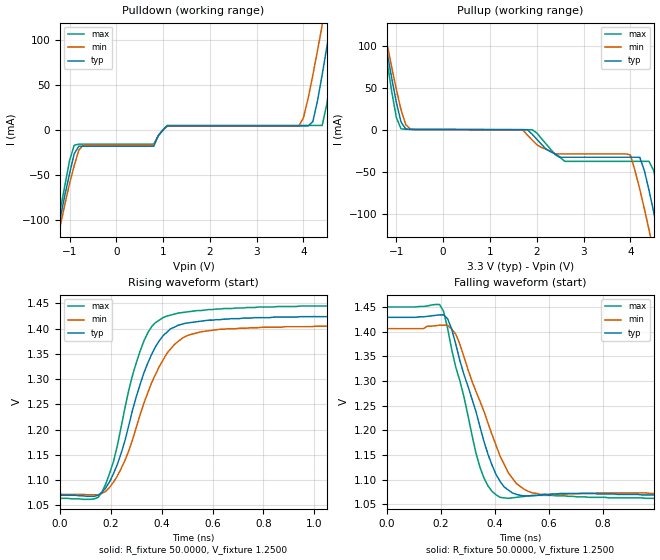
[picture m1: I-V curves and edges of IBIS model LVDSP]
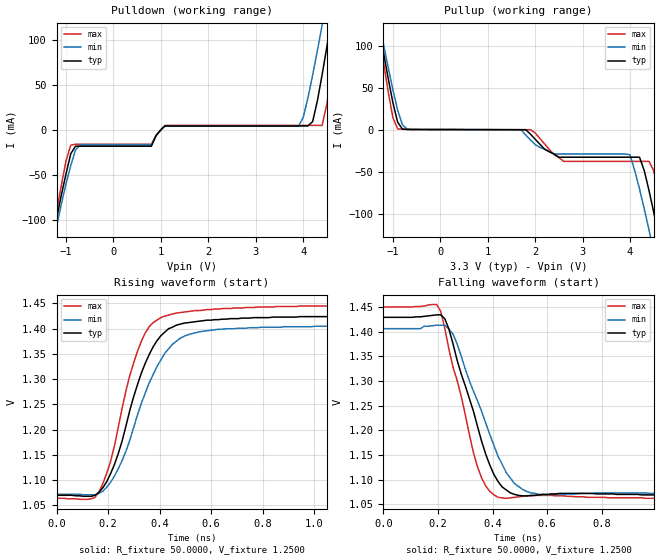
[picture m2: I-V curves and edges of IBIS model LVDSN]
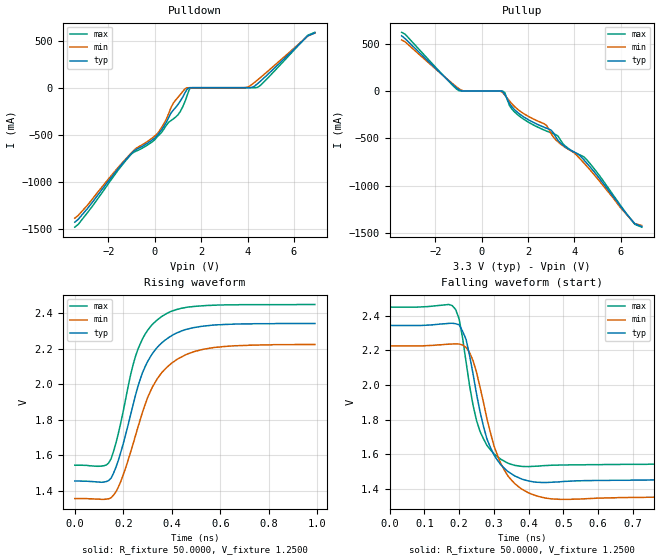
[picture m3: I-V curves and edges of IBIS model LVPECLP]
|   National Semiconductor Corporation
|   IBIS Model of LMK01000
[IBIS Ver]   3.2
[File name]   lmk01000.ibs
[File Rev]   1.1
[Notes] Created by Pegah Alavi
   Rev1.0 : Initial Release
   Rev1.1 : Fixed syntax issues with package model
   (removed spaces in name)
[Date]   04/06/2009
[Source]
[Disclaimer]
(C) Copyright National Semiconductor Corporation 2009
   All rights reserved
National Semiconductor Corporation hereby grants the
user of this IBIS model a non-exclusive, nontransferable
license to use this IBIS model under the following terms.
Before using this IBIS model, the user should read this
license.  If the user does not accept these terms,  the
IBIS model should be returned to National within 30 days.
The user is granted this license only to use the
IBIS model and is not granted rights to sell, load, rent,
lease or license the IBIS model in whole or in part, or in
modified form to anyone other than user. User may modify
the IBIS model to suit its specific applications but rights
to derivative works and such modifications shall belong to
National.
This IBIS model is provided on an "AS IS" basis and
National makes absolutely no warranty with respect to the
information contained herein.NATIONAL DISCLAIMS AND CUSTOMER
WAIVES ALL WARRANTIES, EXPRESS OR IMPLIED, INCLUDING
WARRANTIES OF MERCHANTABILITY OR FITNESS FOR A PARTICULAR
PURPOSE. The entire risk as to quality and performance is
with the Customer. ACCORDINGLY, IN NO EVENT SHALL THE
COMPANY BE LIABLE FOR ANY DAMAGES, WHETHER IN CONTRACT OR
TORT,INCLUDING ANY LOST PROFITS OR OTHER INCIDENTAL,
CONSEQUENTIAL, EXEMPLARY, OR PUNITIVE DAMAGES ARISING OUT
OF THE USE OR APPLICATION OF THE IBIS model provided in
this package.Further, National reserves the right to make
changes without notice to any product herein to improve
reliability, function, or design. National does not convey
any license under patent rights or any other intellectual
property rights, including those of third parties.
National is not obligated to provide maintenance or support
for the licensed IBIS model.
[Copyright]  Copyright 2009, National Semiconductor, All Rights Reserved
[Component]  LMK01000
[Manufacturer]  National Semiconductor Corp
[Package]
|   typ   min   max
R_pkg   0.693   0.432   0.954
L_pkg   1.875nH   1.120nH   2.630nH
C_pkg   0.046pF   0.037pF   0.055pF
[Pin]   signal_name   model_name   R_pin   L_pin   C_pin
1   GND   GND   0.856   2.350nH   0.055pF
2   NC   NC   0.769   2.080nH   0.042pF
3   Vcc1   POWER   0.732   1.960nH   0.040pF
4   CLKuWire   NC   0.71   1.890nH   0.040pF
5   DATAuWire   NC   0.701   1.860nH   0.040pF
6   LEuWire   NC   0.711   1.890nH   0.039pF
7   NC   NC   0.712   1.850nH   0.045pF
8   VCC2   POWER   0.806   2.150nH   0.040pF
9   NC   NC   0.736   1.850nH   0.042pF
10   NC   NC   0.718   1.910nH   0.041pF
11   GOE   NC   0.719   1.940nH   0.041pF
12   TEST   NC   0.751   2.080nH   0.055pF
13   VCC3   POWER   0.736   2.070nH   0.051pF
14   CLKout0   LVDSP   0.715   1.970nH   0.040pF
15   CLKout0*   LVDSN   0.637   1.730nH   0.039pF
16   VCC4   POWER   0.601   1.620nH   0.038pF
17   CLKout1   LVDSP   0.533   1.410nH   0.037pF
18   CLKout1*   LVDSN   0.475   1.240nH   0.037pF
19   VCC5   POWER   0.447   1.160nH   0.037pF
20   CLKout2   LVDSP   0.432   1.120nH   0.038pF
21   CLKout2*   LVDSN   0.442   1.140nH   0.038pF
22   VCC6   POWER   0.465   1.220nH   0.038pF
23   CLKout3   LVPECLP   0.488   1.300nH   0.039pF
24   CLKout3*   LVPECLN   0.542   1.490nH   0.050pF
25   GND   GND   0.666   1.850nH   0.053pF
26   VCC7   POWER   0.580   1.550nH   0.041pF
27   SYNC*   NC   0.508   1.330nH   0.039pF
28   CLKIN0   CLKIN0P   0.469   1.220nH   0.039pF
29   CLKIN0*   CLKIN0N   0.447   1.160nH   0.039pF
30   VCC8   POWER   0.442   1.130nH   0.038pF
31   VCC9   POWER   0.467   1.160nH   0.040pF
32   NC   NC   0.461   1.200nH   0.039pF
33   VCC10   POWER   0.488   1.270nH   0.039pF
34   CLKIN1   CLKIN1P   0.526   1.390nH   0.039pF
35   CLKIN1*   CLKIN1N   0.593   1.580nH   0.041pF
36   BIAS   POWER   0.658   1.810nH   0.053pF
37   VCC11   POWER   0.677   1.880nH   0.051pF
38   CLKout4   LVPECLP   0.666   1.800nH   0.040pF
39   CLKout4*   LVPECLN   0.630   1.670nH   0.038pF
40   VCC12   POWER   0.613   1.620nH   0.039pF
41   CLKout5   LVPECLP   0.611   1.610nH   0.038pF
42   CLKout5*   LVPECLN   0.634   1.680nH   0.038pF
43   VCC13   POWER   0.663   1.760nH   0.038pF
44   CLKout6   LVPECLP   0.701   1.870nH   0.038pF
45   CLKout6*   LVPECLN   0.765   2.040nH   0.038pF
46   VCC14   POWER   0.817   2.190nH   0.039pF
47   CLKout7   LVPECLP   0.874   2.370nH   0.039pF
48   CLKout7*   LVPECLN   0.954   2.630nH   0.051pF
49   DAP   NC
[Diff pin]  inv_pin  vdiff  tdelay_typ  tdelay_min  tdelay_max
14 15   0.0V   0.0s   0.0s   0.0s
17 18   0.0V   0.0s   0.0s   0.0s
20 21   0.0V   0.0s   0.0s   0.0s
23 24   0.0V   0.0s   0.0s   0.0s
28 29   200mV   0.0s   0.0s   0.0s
34 35   200mV   0.0s   0.0s   0.0s
38 39   0.0V   0.0s   0.0s   0.0s
41 42   0.0V   0.0s   0.0s   0.0s
44 45   0.0V   0.0s   0.0s   0.0s
47 48   0.0V   0.0s   0.0s   0.0s
[Define Package Model]  48_LLP
[Manufacturer]   National Semiconductor Corporation
[OEM]   NA
[Description]   48 LLP for LMK01000ISQ, full model
[Number Of Pins]   49
[Pin Numbers]
   1   |   1 = 1
   2   |   2 = 2
   3   |   3 = 3
   4   |   4 = 4
   5   |   5 = 5
   6   |   6 = 6
   7   |   7 = 7
   8   |   8 = 8
   9   |   9 = 9
  10   |  10 = 10
  11   |  11 = 11
  12   |  12 = 12
  13   |  13 = 13
  14   |  14 = 14
  15   |  15 = 15
  16   |  16 = 16
  17   |  17 = 17
  18   |  18 = 18
  19   |  19 = 19
  20   |  20 = 20
  21   |  21 = 21
  22   |  22 = 22
  23   |  23 = 23
  24   |  24 = 24
  25   |  25 = 25
  26   |  26 = 26
  27   |  27 = 27
  28   |  28 = 28
  29   |  29 = 29
  30   |  30 = 30
  31   |  31 = 31
  32   |  32 = 32
  33   |  33 = 33
  34   |  34 = 34
  35   |  35 = 35
  36   |  36 = 36
  37   |  37 = 37
  38   |  38 = 38
  39   |  39 = 39
  40   |  40 = 40
  41   |  41 = 41
  42   |  42 = 42
  43   |  43 = 43
  44   |  44 = 44
  45   |  45 = 45
  46   |  46 = 46
  47   |  47 = 47
  48   |  48 = 48
  49   |  49 = DAP
[Model Data]
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[End Model Data]
[End Package Model]
| Models and submodels in the file (8): LVDSP (Output), LVDSN (Output), LVPECLP (Output), LVPECLN (Output), CLKIN0P (Input), CLKIN0N (Input), CLKIN1P (Input), CLKIN1N (Input)
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|   Model LVDSP
[Model]  LVDSP
Model_type Output
Polarity   Non-Inverting
Vmeas =  1.2780V
Rref =   50.0000
Vref =   1.2500V
C_comp   1.6000pF   1.6000pF   1.6000pF
[Temperature Range]   25.0000   85.0000   -40.0000
[Voltage Range]   3.3000V   3.1500V   3.4500V
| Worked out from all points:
|   slope of the pullup table from 0 to 0.495 V, typ, clamps not added: 9.98 kohm
|   rising waveform, R_fixture 50.0000, V_fixture 1.2500: 20-80 % time 134ps typ, 152ps min, 115ps max; typ from 1.07 V to 1.43 V
|   falling waveform, R_fixture 50.0000, V_fixture 1.2500: 20-80 % time 119ps typ, 137ps min, 101ps max; typ from 1.43 V to 1.07 V
[Pulldown]
|Voltage   I(typ)   I(min)   I(max)
-3.45V    -669.4mA   -638.7mA   -724mA
-1.3V     -126.3mA   -133.2mA   -120mA
-900mV    -26.71mA   -39.95mA   -17.23mA
-700mV    -18.3mA    -16.89mA   -16.07mA
800mV     -18.3mA    -16.89mA   -16.07mA
1.1V      4.237mA    3.877mA    4.82mA
3.9V      4.237mA    3.877mA    4.82mA
4.2V      9.056mA    60.8mA     4.82mA
4.4V      61.28mA    116.4mA    4.82mA
4.6V      124.2mA    174mA      63.07mA
4.8V      189.4mA    232.6mA    137mA
6.9V      832.6mA    800.9mA    875.6mA
[Pullup]
|Voltage   I(typ)   I(min)   I(max)
-3.45V    832.6mA    755.7mA    934.3mA
-1.3V     124.2mA    130.7mA    118.2mA
-900mV    9.056mA    23.5mA     1.096mA
-700mV    356.2uA    687.6uA    401.7uA
1.9V      -5.159mA   -12.12mA   33.99uA
2.6V      -32.65mA   -28.75mA   -37.57mA
4V        -32.65mA   -29.82mA   -37.57mA
4.2V      -32.65mA   -70.34mA   -37.57mA
4.4V      -72.21mA   -119.1mA   -37.57mA
4.6V      -125.3mA   -170.8mA   -75.8mA
4.8V      -181.4mA   -223.8mA   -134.7mA
6.9V      -666.4mA   -669.2mA   -681mA
[Ramp]
| variable   typ   min   max
dV/dt_r  0.2150/0.1345n   0.2004/0.1510n   0.2300/0.1137n
dV/dt_f  0.2172/0.1181n   0.2037/0.1385n   0.2318/0.1004n
R_load = 50.00
[Rising Waveform]
R_fixture= 50.0000
V_fixture= 1.2500
V_fixture_min= 1.2500
V_fixture_max= 1.2500
|time   V(typ)   V(min)   V(max)
0s        1.07V      1.072V     1.064V
165ps     1.076V     1.074V     1.077V
225ps     1.131V     1.108V     1.168V
270ps     1.208V     1.158V     1.278V
315ps     1.29V      1.23V      1.356V
360ps     1.349V     1.293V     1.404V
405ps     1.386V     1.338V     1.422V
480ps     1.409V     1.381V     1.432V
630ps     1.418V     1.399V     1.439V
1.485ns   1.426V     1.406V     1.448V
[Falling Waveform]
R_fixture= 50.0000
V_fixture= 1.2500
V_fixture_min= 1.2500
V_fixture_max= 1.2500
|time   V(typ)   V(min)   V(max)
0s        1.429V     1.406V     1.45V
195ps     1.434V     1.413V     1.455V
225ps     1.426V     1.413V     1.406V
255ps     1.375V     1.395V     1.328V
345ps     1.207V     1.259V     1.125V
375ps     1.151V     1.214V     1.087V
420ps     1.096V     1.147V     1.064V
480ps     1.07V      1.092V     1.064V
570ps     1.069V     1.07V      1.068V
1.485ns   1.069V     1.071V     1.06V
|   Model LVDSN
[Model]  LVDSN
Model_type Output
Polarity   Inverting
Vmeas =  1.2780V
Rref =   50.0000
Vref =   1.2500V
C_comp   1.6000pF   1.60000pF   1.60000pF
[Temperature Range]   25.0000   85.0000   -40.0000
[Voltage Range]   3.3000V   3.1500V   3.4500V
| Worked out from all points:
|   slope of the pullup table from 0 to 0.495 V, typ, clamps not added: 9.98 kohm
|   rising waveform, R_fixture 50.0000, V_fixture 1.2500: 20-80 % time 134ps typ, 152ps min, 115ps max; typ from 1.07 V to 1.43 V
|   falling waveform, R_fixture 50.0000, V_fixture 1.2500: 20-80 % time 119ps typ, 137ps min, 101ps max; typ from 1.43 V to 1.07 V
[Pulldown]
|Voltage   I(typ)   I(min)   I(max)
-3.45V    -669.4mA   -638.7mA   -724mA
-1.3V     -126.3mA   -133.2mA   -120mA
-900mV    -26.71mA   -39.95mA   -17.23mA
-700mV    -18.3mA    -16.89mA   -16.07mA
800mV     -18.3mA    -16.89mA   -16.07mA
1.1V      4.237mA    3.877mA    4.82mA
3.9V      4.237mA    3.877mA    4.82mA
4.2V      9.056mA    60.8mA     4.82mA
4.4V      61.28mA    116.4mA    4.82mA
4.6V      124.2mA    174mA      63.07mA
4.8V      189.4mA    232.6mA    137mA
6.9V      832.6mA    800.9mA    875.6mA
[Pullup]
|Voltage   I(typ)   I(min)   I(max)
-3.45V    832.6mA    755.7mA    934.3mA
-1.3V     124.2mA    130.7mA    118.2mA
-900mV    9.056mA    23.5mA     1.096mA
-700mV    356.2uA    687.6uA    401.7uA
1.9V      -5.159mA   -12.12mA   33.99uA
2.6V      -32.65mA   -28.75mA   -37.57mA
4V        -32.65mA   -29.82mA   -37.57mA
4.2V      -32.65mA   -70.34mA   -37.57mA
4.4V      -72.21mA   -119.1mA   -37.57mA
4.6V      -125.3mA   -170.8mA   -75.8mA
4.8V      -181.4mA   -223.8mA   -134.7mA
6.9V      -666.4mA   -669.2mA   -681mA
[Ramp]
| variable   typ   min   max
dV/dt_r  0.2150/0.1345n   0.2004/0.1510n   0.2300/0.1137n
dV/dt_f  0.2172/0.1181n   0.2037/0.1385n   0.2318/0.1004n
R_load = 50.00
[Rising Waveform]
R_fixture= 50.0000
V_fixture= 1.2500
V_fixture_min= 1.2500
V_fixture_max= 1.2500
|time   V(typ)   V(min)   V(max)
0s        1.07V      1.072V     1.064V
165ps     1.076V     1.074V     1.077V
225ps     1.131V     1.108V     1.168V
270ps     1.208V     1.158V     1.278V
315ps     1.29V      1.23V      1.356V
360ps     1.349V     1.293V     1.404V
405ps     1.386V     1.338V     1.422V
480ps     1.409V     1.381V     1.432V
630ps     1.418V     1.399V     1.439V
1.485ns   1.426V     1.406V     1.448V
[Falling Waveform]
R_fixture= 50.0000
V_fixture= 1.2500
V_fixture_min= 1.2500
V_fixture_max= 1.2500
|time   V(typ)   V(min)   V(max)
0s        1.429V     1.406V     1.45V
195ps     1.434V     1.413V     1.455V
225ps     1.426V     1.413V     1.406V
255ps     1.375V     1.395V     1.328V
345ps     1.207V     1.259V     1.125V
375ps     1.151V     1.214V     1.087V
420ps     1.096V     1.147V     1.064V
480ps     1.07V      1.092V     1.064V
570ps     1.069V     1.07V      1.068V
1.485ns   1.069V     1.071V     1.06V
|   Model LVPECLP
[Model]  LVPECLP
Model_type Output
Polarity   Non-Inverting
Vmeas =  1.9400V
Rref =   50.0000
Vref =   1.2500V
C_comp   1.1000pF   1.1000pF   1.100pF
[Temperature Range]   25.0000   85.0000   -40.0000
[Voltage Range]   3.3000V   3.1500V   3.4500V
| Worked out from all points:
|   slope of the pulldown table from 0 to 0.495 V, typ, clamps not added: 2.95 ohm
|   rising waveform, R_fixture 50.0000, V_fixture 1.2500: 20-80 % time 123ps typ, 140ps min, 104ps max; typ from 1.46 V to 2.34 V
|   falling waveform, R_fixture 50.0000, V_fixture 1.2500: 20-80 % time 61.3ps typ, 72ps min, 51.6ps max; typ from 2.34 V to 1.45 V
[Pulldown]
|Voltage   I(typ)   I(min)   I(max)
-3.45V    -1.429A    -1.387A    -1.482A
-1.1V     -722.9mA   -716.3mA   -729.3mA
100mV     -509.2mA   -491.3mA   -523.3mA
400mV     -409mA     -379.8mA   -437mA
800mV     -237.4mA   -162.8mA   -331.3mA
1V        -178mA     -102.2mA   -287.5mA
1.2V      -101.2mA   -41.1mA    -204.8mA
1.5V      -613.3uA   -58.5uA    -11.3mA
3.9V      173.5nA    754.6uA    57.2pA
4.4V      36.18mA    76.19mA    1.372mA
6.6V      551.6mA    550.5mA    558.3mA
6.9V      581.6mA    580.5mA    588.3mA
[Pullup]
|Voltage   I(typ)   I(min)   I(max)
-3.45V    581.6mA    537.7mA    618.2mA
-1V       16.83mA    27.74mA    5.801mA
900mV     -5.507mA   -15.29mA   -325.7uA
1V        -38.16mA   -43.45mA   -19.47mA
1.2V      -130.1mA   -105.9mA   -154.5mA
1.5V      -215.9mA   -182.5mA   -239.6mA
2.8V      -392.6mA   -364.2mA   -422.4mA
3.2V      -486.7mA   -515.5mA   -460.3mA
3.6V      -587.8mA   -594.2mA   -579.3mA
4.5V      -751.4mA   -783.9mA   -716.1mA
6.6V      -1.398A    -1.397A    -1.405A
6.9V      -1.428A    -1.417A    -1.435A
[Ramp]
| variable   typ   min   max
dV/dt_r  0.5335/0.1232n   0.5233/0.1420n   0.5443/0.1040n
dV/dt_f  0.5335/0.0610n   0.5220/0.0720n   0.5452/0.0514n
R_load = 50.0000
[Rising Waveform]
R_fixture= 50.0000
V_fixture= 1.2500
V_fixture_min= 1.2300
V_fixture_max= 1.2700
|time   V(typ)   V(min)   V(max)
0s        1.455V     1.356V     1.544V
140ps     1.458V     1.355V     1.557V
190ps     1.618V     1.454V     1.785V
230ps     1.827V     1.617V     2.051V
260ps     1.985V     1.756V     2.195V
300ps     2.126V     1.923V     2.302V
360ps     2.234V     2.067V     2.382V
430ps     2.293V     2.146V     2.423V
550ps     2.329V     2.201V     2.443V
990ps     2.341V     2.223V     2.448V
[Falling Waveform]
R_fixture= 50.0000
V_fixture= 1.2500
V_fixture_min= 1.2300
V_fixture_max= 1.2700
|time   V(typ)   V(min)   V(max)
0s        2.343V     2.225V     2.449V
170ps     2.355V     2.235V     2.464V
200ps     2.347V     2.236V     2.38V
220ps     2.262V     2.216V     2.131V
240ps     2.063V     2.14V      1.883V
260ps     1.847V     1.988V     1.732V
300ps     1.597V     1.65V      1.603V
340ps     1.501V     1.476V     1.549V
470ps     1.439V     1.342V     1.537V
990ps     1.454V     1.355V     1.544V
